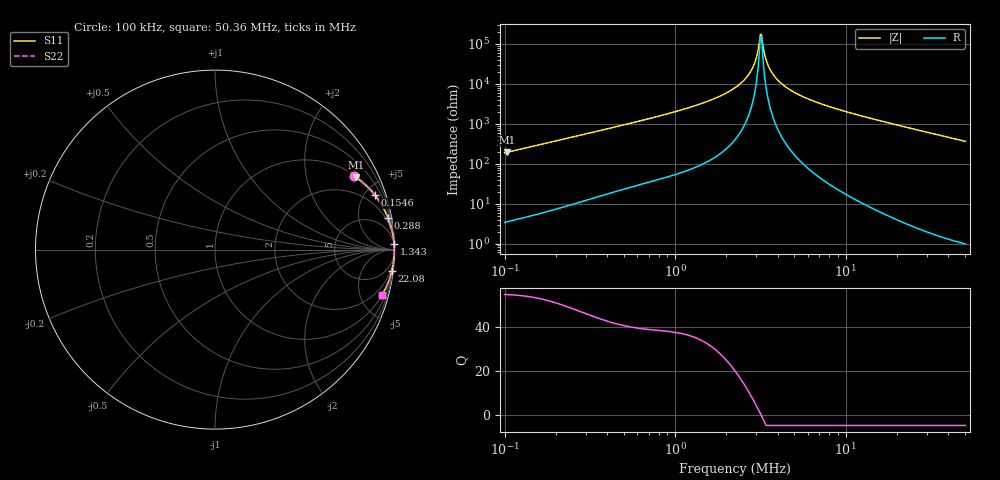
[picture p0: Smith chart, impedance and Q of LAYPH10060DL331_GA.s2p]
! LAYPH10060DL331_GA  S-PARAMETER MODEL  ( General Type )
! Model Generated by TAIYO YUDEN Corporation (http://www.ty-top.com)
! Version 3.0
! TAIYO YUDEN Control No. 180828NI43SB-FBB
! Copyright(c) 2017 TAIYO YUDEN CO.,LTD. All Rights Reserved.
! Product Description (link to TY-COMPAS)
! https://ds.yuden.co.jp/TYCOMPAS/or/detail?pn=LAYPH10060DL331MGA&u=M
! Products Name : Inductors
! Characteristics :
!  Inductance : 330 uH , SRF(min) : -Hz , DC Resistance(max) : 0.55 Ohm
!  Rated Current : Saturation :0.75 A , Temp Rise : 0.58 A (25 degC)
!  Case Size : 10.1 x 10.0 / 0.398 x 0.394 [mm/inch] , Thickness : 6 / 0.236 [mm/inch]
!  (Conditions: Temperature = 25 degC , DC Bias Current/Voltage = 0A / 0V)
! External Node Assignments :
!  1  o---GGG---o  2
! GND o---------o GND
! Frequency Range : 0.1MHz  -  50.361429MHz  [ 402 STEP ]
# MHz S RI R 50
! Freq[MHz].  S11 Real  S11 Imag  S21 Real  S21 Imag  S12 Real  S12 Imag  S22 Real  S22 Imag
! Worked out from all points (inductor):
!   401 points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, 100 kHz to 50.36 MHz, reference 50 ohm
!   read as one part in series: L = 298 uH near 103.2 kHz
!   highest Q = 55.1 at 103.2 kHz (marker M1), where L = 299 uH
!   self-resonance near 3.16 MHz
!   S11 on the Smith chart (normalised r, x): 100 kHz: 1.07, +3.75; 154.6 kHz: 1.11, +5.79; 288 kHz: 1, +11; 1.343 MHz: 3, +59; 22.08 MHz: 1, -17; 50.36 MHz: 1.02, -7.29
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0.1  0.7747 0.4088  0.2253 -0.4088  0.2253 -0.4088  0.7747 0.4088
0.10316  0.7851 0.4018  0.2149 -0.4018  0.2149 -0.4018  0.7851 0.4018
0.154578  0.8888 0.3051  0.1112 -0.3051  0.1112 -0.3051  0.8888 0.3051
0.283532  0.9621 0.1806  0.0379 -0.1806  0.0379 -0.1806  0.9621 0.1806
0.287976  0.9631 0.178  0.0369 -0.178  0.0369 -0.178  0.9631 0.178
0.803902  0.9943 0.0633  0.00568 -0.0633  0.00568 -0.0633  0.9943 0.0633
1.343154  0.9979 0.0336  0.0021 -0.0336  0.0021 -0.0336  0.9979 0.0336
1.833289  0.9989 0.0201  0.00113 -0.0201  0.00113 -0.0201  0.9989 0.0201
2.279315  0.9992 0.0118  0.000751 -0.0118  0.000751 -0.0118  0.9992 0.0118
2.581346  0.9994 0.00734  0.000619 -0.00734  0.000619 -0.00734  0.9994 0.00734
2.790117  0.9994 0.0046  0.000563 -0.0046  0.000563 -0.0046  0.9994 0.0046
2.969227  0.9995 0.00243  0.000531 -0.00243  0.000531 -0.00243  0.9995 0.00243
3.111066  0.9995 0.000807  0.000514 -0.000807  0.000514 -0.000807  0.9995 0.000807
3.209369  0.9995 -0.000274  0.000506 0.000274  0.000506 0.000274  0.9995 -0.000274
3.25968  0.9995 -0.000814  0.000504 0.000814  0.000504 0.000814  0.9995 -0.000814
3.523312  0.9995 -0.00352  0.0005 0.00352  0.0005 0.00352  0.9995 -0.00352
3.9286  0.9995 -0.00735  0.000524 0.00735  0.000524 0.00735  0.9995 -0.00735
4.734791  0.9994 -0.0142  0.000647 0.0142  0.000647 0.0142  0.9994 -0.0142
6.362832  0.9989 -0.026  0.0011 0.026  0.0011 0.026  0.9989 -0.026
18.04064  0.9905 -0.0946  0.00947 0.0946  0.00947 0.0946  0.9905 -0.0946
22.08361  0.9858 -0.1165  0.0142 0.1165  0.0142 0.1165  0.9858 -0.1165
50.36143  0.9295 -0.2547  0.0705 0.2547  0.0705 0.2547  0.9295 -0.2547
